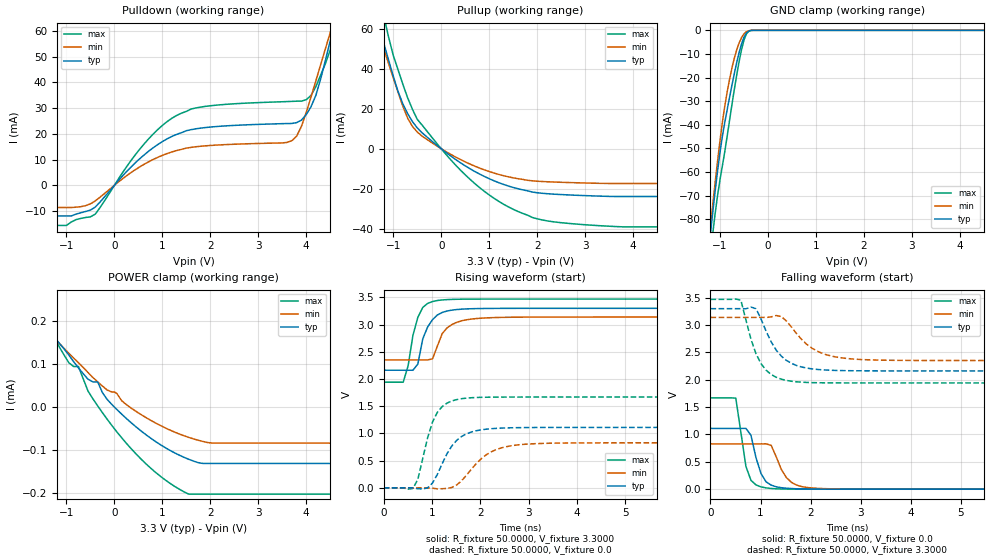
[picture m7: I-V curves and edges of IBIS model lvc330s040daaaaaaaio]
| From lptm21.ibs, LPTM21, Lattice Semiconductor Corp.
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|   Model lvc330s040daaaaaaaio
[Model]   lvc330s040daaaaaaaio
Model_type   I/O
Polarity   Non-Inverting
Enable   Active-Low
Vinl =   0.8000V
Vinh =   2.0000V
Vmeas =   1.500000V
Cref =   0.0F
Rref =   1.0000M
Vref =   0.0V
C_comp   4.2000pF   3.8000pF   7.5000pF
[Temperature Range]   25.0000   0.1050k   -40.0000
[Voltage Range]   3.3000V   3.1400V   3.4700V
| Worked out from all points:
|   slope of the pulldown table from 0 to 0.495 V, typ, clamps not added: 50.7 ohm
|   slope of the pullup table from 0 to 0.495 V, typ, clamps not added: 58.5 ohm
|   GND clamp passes 1 mA (typ) near -0.44 V on its own axis
|   rising waveform, R_fixture 50.0000, V_fixture 3.3000: 20-80 % time 264ps typ, 311ps min, 218ps max; typ from 2.16 V to 3.3 V
|   rising waveform, R_fixture 50.0000, V_fixture 0.0: 20-80 % time 438ps typ, 579ps min, 327ps max; typ from 0 V to 1.11 V
|   falling waveform, R_fixture 50.0000, V_fixture 0.0: 20-80 % time 219ps typ, 291ps min, 181ps max; typ from 1.11 V to 0 V
|   falling waveform, R_fixture 50.0000, V_fixture 3.3000: 20-80 % time 443ps typ, 565ps min, 361ps max; typ from 3.3 V to 2.16 V
[Pulldown]
|Voltage   I(typ)   I(min)   I(max)
-3.3V     -11.92mA   -8.642mA   -15.6mA
-1V       -11.92mA   -8.642mA   -15.6mA
-500mV    -9.624mA   -7.225mA   -12.27mA
600mV     11.49mA    7.938mA    15.62mA
1.3V      19.78mA    13.49mA    27.13mA
2V        22.6mA     15.45mA    30.87mA
3.7V      23.99mA    17.3mA     32.57mA
3.9V      25.28mA    22.85mA    32.67mA
4.1V      30.47mA    34.23mA    34.88mA
4.5V      56mA       59.18mA    52.45mA
4.6V      63.61mA    65.35mA    60.64mA
6.6V      186.4mA    170.2mA    211.9mA
[Pullup]
|Voltage   I(typ)   I(min)   I(max)
-3.3V     181.6mA    129.5mA    218.7mA
-1.4V     69.53mA    64.71mA    88.1mA
-1.3V     61.25mA    57.43mA    77.39mA
-1.2V     52.87mA    50.1mA     66.58mA
-1.1V     44.47mA    42.74mA    55.99mA
-800mV    22.38mA    21.23mA    32.17mA
-500mV    10.43mA    8.389mA    14.69mA
600mV     -9.992mA   -7.668mA   -15.26mA
1.6V      -19.98mA   -14.96mA   -31.34mA
2.2V      -22.45mA   -16.49mA   -36.01mA
3.2V      -23.59mA   -17.23mA   -38.3mA
6.55V     -23.86mA   -17.35mA   -39.03mA
[GND_clamp]
|Voltage   I(typ)   I(min)   I(max)
-3.3V     -955.2mA   -930.2mA   -977.8mA
-1.2V     -86.08mA   -82.87mA   -94.74mA
-1.15V    -76.63mA   -73.22mA   -85.57mA
-1.1V     -67.6mA    -63.89mA   -77.12mA
-1V       -51.41mA   -46.51mA   -63.06mA
-900mV    -38.77mA   -31.82mA   -51.11mA
-800mV    -28.16mA   -20.53mA   -37.82mA
-700mV    -18.01mA   -11.58mA   -24.66mA
-600mV    -9.185mA   -5.219mA   -12.92mA
-450mV    -1.125mA   -553.6uA   -1.501mA
-300mV    0A         0A         0A
6.6V      0A         0A         0A
[POWER_clamp]
|Voltage   I(typ)   I(min)   I(max)
-3.25V    961.3uA    1.05mA     917.9uA
-2.05V    275.4uA    268.3uA    307.1uA
-1.75V    231.3uA    224.8uA    252.6uA
-950mV    120.7uA    124.7uA    102.8uA
-750mV    90.82uA    102.7uA    94.17uA
-450mV    58.57uA    68.87uA    19.46uA
-350mV    58.57uA    58.54uA    3.121uA
50mV      -5.338uA   31.71uA    -57.16uA
850mV     -79.07uA   -36.24uA   -150.4uA
1.55V     -120.8uA   -70.05uA   -201.6uA
2.05V     -130.5uA   -83.29uA   -201.6uA
6.6V      -130.5uA   -83.29uA   -201.6uA
[Ramp]
| variable   typ   min   max
dV/dt_r  0.7026/0.4330n   0.4966/0.5731n   1.0018/0.3242n
dV/dt_f  0.6827/0.4387n   0.4730/0.5599n   0.9168/0.3576n
R_load = 50.0000
[Rising Waveform]
R_fixture=   50.0000
V_fixture=   3.3000
V_fixture_min=   3.1400
V_fixture_max=   3.4700
|time   V(typ)   V(min)   V(max)
0s        2.162V     2.352V     1.942V
404ps     2.162V     2.352V     1.942V
606.1ps   2.162V     2.352V     2.806V
707.1ps   2.276V     2.352V     3.134V
808.1ps   2.736V     2.352V     3.316V
1.01ns    3.091V     2.37V      3.424V
1.111ns   3.177V     2.605V     3.443V
1.414ns   3.267V     3.002V     3.464V
2.02ns    3.296V     3.119V     3.47V
10ns      3.3V       3.14V      3.47V
[Rising Waveform]
R_fixture=   50.0000
V_fixture=   0.0
V_fixture_min=   0.0
V_fixture_max=   0.0
|time   V(typ)   V(min)   V(max)
0s        1.288uV    1.554uV    1.323uV
606.1ps   -395.5uV   2.808uV    -9.94mV
707.1ps   -15.72mV   17.67uV    156.1mV
909.1ps   -458.6uV   -207.2uV   922.6mV
1.01ns    88.34mV    -6.184mV   1.209V
1.212ns   447.1mV    -16.04mV   1.495V
1.515ns   876.6mV    55.59mV    1.623V
2.121ns   1.079V     606.6mV    1.666V
2.828ns   1.107V     794.2mV    1.669V
10ns      1.111V     827.7mV    1.67V
[Falling Waveform]
R_fixture=   50.0000
V_fixture=   0.0
V_fixture_min=   0.0
V_fixture_max=   0.0
|time   V(typ)   V(min)   V(max)
0s        1.111V     827.7mV    1.67V
505.1ps   1.111V     827.7mV    1.664V
707.1ps   1.111V     827.7mV    415.7mV
808.1ps   985.1mV    827.7mV    161.2mV
1.01ns    281.4mV    828.2mV    40.87mV
1.111ns   132.9mV    828.5mV    22.94mV
1.212ns   73.68mV    799.7mV    12.45mV
1.515ns   17.1mV     211.6mV    2.151mV
2.02ns    2.152mV    21.8mV     239.2uV
10ns      -1.071uV   8.416uV    -6.671uV
[Falling Waveform]
R_fixture=   50.0000
V_fixture=   3.3000
V_fixture_min=   3.1400
V_fixture_max=   3.4700
|time   V(typ)   V(min)   V(max)
0s        3.3V       3.14V      3.47V
606.1ps   3.3V       3.14V      3.457V
808.1ps   3.33V      3.14V      2.74V
909.1ps   3.299V     3.14V      2.475V
1.01ns    3.108V     3.141V     2.293V
1.212ns   2.692V     3.151V     2.097V
1.515ns   2.355V     3.075V     1.988V
2.02ns    2.2V       2.581V     1.948V
2.727ns   2.167V     2.389V     1.942V
10ns      2.162V     2.352V     1.942V
